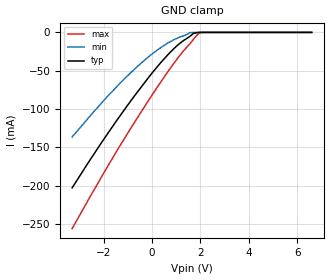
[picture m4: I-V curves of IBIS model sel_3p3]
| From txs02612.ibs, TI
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|   sel_3p3 Model
[Model]   sel_3p3
Model_type   Input
Vinl = 1.155
Vinh = 2.145
|   typ   min   max
|   (nom PVT)   (fast PVT)   (slow PVT)
|C_comp from frequency sweep method (F=60MHz)
|Average
|C_comp   1.626e-11   1.513e-11   1.851e-11
|C_comp from LC tank measurement(L=1nH)
|Average
|Resonant Frequency(Hz)   3.760e+09   4.100e+09   3.660e+09
C_comp   1.793e-12   1.508e-12   1.893e-12
[Model spec]
|subparameter
Vinl   1.155   1.05   1.26
Vinh   2.145   1.95   2.34
| Where nom  PVT is Nominal Process, 3.3V, 27C
|   Fast PVT is Strong Process,  3.6V, -40C
|   Slow PVT is Weak Process,   3V, 125C
[Voltage Range]   3.3   3   3.6
|Ambient Temperature   25   85   -40
|Junction Temperature
[Temperature Range]   27   125   -40
[Power Clamp Reference]   3.3   3   3.6
[GND Clamp Reference]   0   0   0
[GND Clamp]
|   Voltage   I(typ)   I(min)   I(max)
-3.3V     -202.7mA   -136.3mA   -255.9mA
-2.424V   -159.9mA   -104mA     -207mA
-1.383V   -111.5mA   -68.3mA    -150.9mA
-591mV    -77.28mA   -44.09mA   -110.7mA
-132mV    -58.33mA   -31.57mA   -88.16mA
633mV     -29.88mA   -14.25mA   -52.22mA
1.092V    -15.75mA   -6.898mA   -32.39mA
1.566V    -5.108mA   -330.3uA   -14.76mA
1.709V    -1.4mA     -142.4uA   -9.153mA
1.94V     -285.9nA   0A         -1.393mA
2.077V    -114.1nA   0A         -8.765uA
6.6V      0A         0A         0A
[POWER Clamp]
|   Voltage   I(typ)   I(min)   I(max)
-3.3V     0A         0A         0A
0V        0A         0A         0A
6.6V      0A         0A         0A
